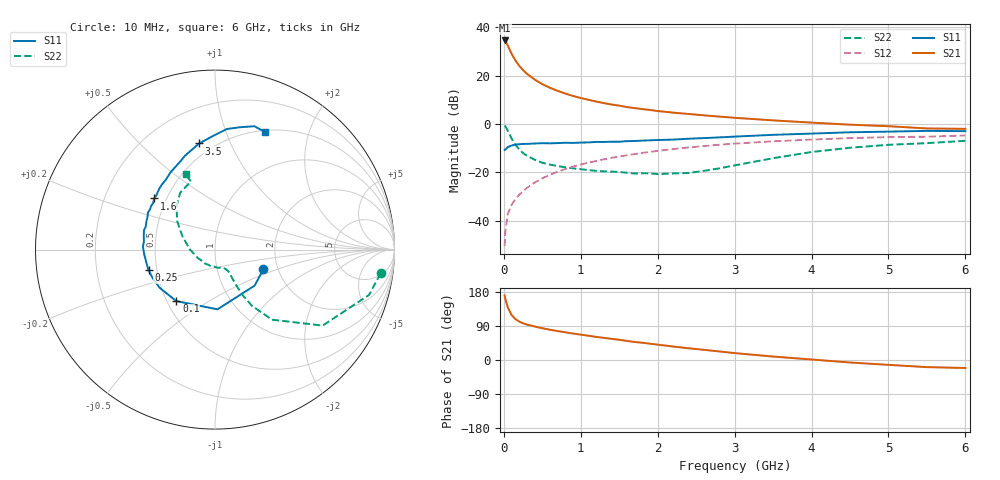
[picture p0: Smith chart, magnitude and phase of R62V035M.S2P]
! SIEMENS Small Signal Semiconductors
! BFR193
! Si NPN RF Bipolar Junction Transistor in SOT23
! VCE = 2 V  IC = 35 mA
! Common Emitter S-Parameters:  May  1996
# GHz  S  MA  R  50
!  f  S11  S21  S12  S22
! GHz  MAG  ANG  MAG  ANG  MAG  ANG  MAG  ANG
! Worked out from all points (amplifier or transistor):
!   36 points, 10 MHz to 6 GHz, reference 50 ohm
!   highest |S21| = 34.5 dB at 10 MHz (marker M1)
!   |S21| within 3 dB of that: start of sweep to 64.24 MHz
!   unconditionally stable (mu >= 1): 430.8 MHz to 1.861 GHz
!   at 250 MHz: K = 0.93, MSG = 25.0 dB, |S12| = -27.8 dB
!   at 1.4 GHz: K = 1.02, MAG = 10.1 dB, |S12| = -14.0 dB
!   at 6 GHz: K = 0.96, MSG = 1.4 dB, |S12| = -4.7 dB
!   S11 on the Smith chart (normalised r, x): 10 MHz: 1.68, -0.41; 100 MHz: 0.56, -0.37; 250 MHz: 0.45, -0.12; 1.6 GHz: 0.43, +0.30; 3.5 GHz: 0.42, +0.77; 6 GHz: 0.52, +1.38
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0.01  0.2913 -22.3  53.17 170.3  0.003 78.1  0.9321 -8.2
0.02  0.2984 -42.3  51.33 161.1  0.006 79.3  0.8945 -16.4
0.05  0.333 -87.6  42.12 139.5  0.0137 69.5  0.7343 -35.2
0.1  0.3587 -126.9  28.39 118.9  0.0213 67.1  0.5031 -50.9
0.15  0.375 -145.7  20.58 108.0  0.0279 67.2  0.3743 -56.7
0.2  0.3821 -155.9  15.96 101.4  0.0345 69.4  0.2997 -58.7
0.25  0.3876 -162.8  12.92 96.8  0.0409 70.4  0.2513 -59.1
0.3  0.3888 -168.2  10.9 93.5  0.0479 72.0  0.2217 -59.2
0.4  0.3957 -176.7  8.293 88.4  0.0617 72.6  0.1836 -59.0
0.5  0.4019 177.8  6.665 83.8  0.0755 72.8  0.1583 -58.1
0.6  0.3987 173.4  5.597 79.9  0.0895 72.3  0.1453 -58.3
0.7  0.4039 169.2  4.84 76.3  0.1036 71.6  0.1357 -59.2
0.8  0.4101 165.0  4.246 73.1  0.1174 70.5  0.1276 -61.0
0.9  0.4069 161.5  3.791 69.8  0.1318 69.4  0.1213 -61.5
1.1  0.4166 154.8  3.159 64.0  0.1593 67.2  0.1118 -67.9
1.3  0.426 148.4  2.704 58.5  0.1868 64.3  0.1053 -73.6
1.6  0.4429 139.9  2.239 50.3  0.2265 60.2  0.0985 -88.0
2.2  0.4766 124.9  1.719 35.6  0.3033 51.2  0.0954 -124.9
3.5  0.598 98.5  1.189 9.1  0.4387 30.5  0.1968 157.6
4.5  0.675 84.4  0.969 -6.6  0.5116 16.3  0.3237 131.4
5.5  0.7216 72.3  0.81 -18.8  0.5459 2.4  0.4029 109.4
6  0.7118 66.9  0.794 -21.1  0.5804 -1.7  0.45 111.4
